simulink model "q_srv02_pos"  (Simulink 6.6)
settings: Solver=ode1  StartTime=0.0  StopTime=inf  FixedStep=0.002  RelTol=1e-3  AbsTol=1e-6
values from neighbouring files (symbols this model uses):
  K_AMP = 1    [setup_srv02_exp02_pos.m]    (also in setup_srv02_exp01_mdl.m; setup_srv02_exp03_spd.m)
  K_ENC = 0    [config_srv02.m]
  K_POT = -(352 * pi / 180 / 10)    (= -0.614355896702)    [config_srv02.m]
  K_TACH = -(1000 * 2 * pi / 60 / 1.5 / Kg)    [config_srv02.m]
  ki = -( -AmpMax + kp * e_ss ) / ti / e_ss    [d_i_design.m]    (also in setup_srv02_exp02_pos.m = 0; d_pi_design.m = wn^2*tau/K; setup_srv02_exp03_spd.m = 0)
  kp = wn^2/K*tau    [d_pv_design.m]    (also in setup_srv02_exp02_pos.m = 0; d_pi_design.m = (-1+2*zeta*wn*tau)/K; setup_srv02_exp03_spd.m = 0)
  kv = (-1+2*zeta*wn*tau)/K    [d_pv_design.m]    (also in setup_srv02_exp02_pos.m = 0)
  VMAX_AMP = 0    [config_srv02.m]
  VMAX_DAC = 10    [setup_srv02_exp02_pos.m]    (also in setup_srv02_exp01_mdl.m; setup_srv02_exp03_spd.m)
  wcf = 2 * pi * 50.0    (= 314.159265359)    [setup_srv02_exp02_pos.m]    (also in setup_srv02_exp03_spd.m)
  wcf_e = 2 * pi * 50.0    (= 314.159265359)    [setup_srv02_exp02_pos.m]    (also in setup_srv02_exp01_mdl.m = 157.079632679; setup_srv02_exp03_spd.m = 395.840674352)
  zetaf = 0.9    [setup_srv02_exp02_pos.m]    (also in setup_srv02_exp03_spd.m)
  zetaf_e = 0.9    [setup_srv02_exp02_pos.m]    (also in setup_srv02_exp01_mdl.m; setup_srv02_exp03_spd.m)
undefined symbols (not defined in the file or in its folder): HIL, qc_get_step_size, square
libraries: quarc_library x5

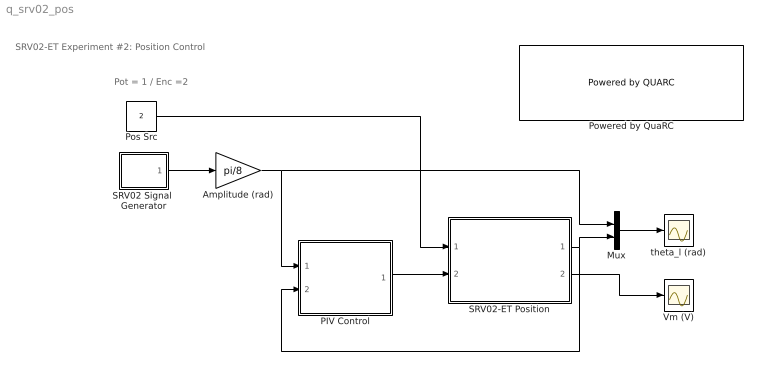
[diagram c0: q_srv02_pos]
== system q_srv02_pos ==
  note: SRV02-ET Experiment #2: Position Control
  note: Pot = 1 / Enc =2
  Amplitude (rad) : Gain  Gain=pi/8
  Mux : Mux  Inputs=2
  PIV Control : Subsystem
  Pos Src : Constant  Value=2
  Powered by QuaRC : quarc_library/Logos/Powered by QUARC  SystemSampleTime=-1
  SRV02 Signal  Generator : Subsystem  mask(QET Signal Generator){sig_type=square, a=1, f=0.4}
      mask prompts: sig_type "Signal Type"; a "Amplitude"; f "Frequency (Hz)"
      mask help: Generates a square, triangular, or sinusoidal waveform of a specified amplitude and frequency.
  SRV02-ET Position : Subsystem
  Vm (V) : Scope
  theta_l (rad) : Scope
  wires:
  Amplitude (rad)/1 -> Mux/1, PIV Control/1(theta_d (rad))
  SRV02-ET Position/1(theta_l (rad)) -> Mux/2, PIV Control/2(theta_l (rad))
  SRV02-ET Position/2(Vm (V)) -> Vm (V)/1
  Mux/1 -> theta_l (rad)/1
  PIV Control/1(u (V)) -> SRV02-ET Position/2(Vi (V))
  SRV02 Signal  Generator/1(out) -> Amplitude (rad)/1
  Pos Src/1 -> SRV02-ET Position/1(pos src)

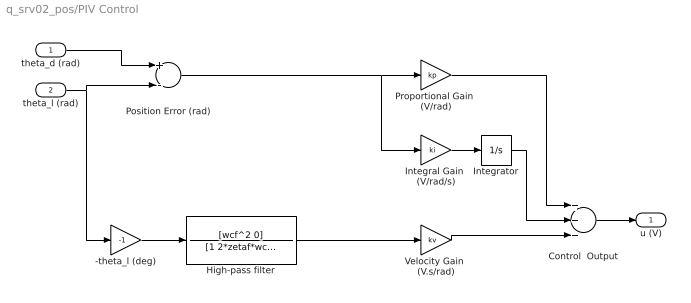
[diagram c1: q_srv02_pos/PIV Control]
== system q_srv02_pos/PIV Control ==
  theta_d (rad) : Inport
  theta_l (rad) : Inport  Port=2
  -theta_l (deg) : Gain  Gain=-1
  Control  Output : Sum  Inputs=+++  OutScaling=2^-10
  High-pass filter : TransferFcn  Numerator=[wcf^2 0]  Denominator=[1 2*zetaf*wcf wcf^2]
  Integral Gain  (V/rad/s) : Gain  Gain=ki
  Integrator : Integrator  LimitOutput=on  UpperSaturationLimit=VMAX_DAC  LowerSaturationLimit=-VMAX_DAC
  Position Error (rad) : Sum  Inputs=+-  OutScaling=2^-10
  Proportional Gain  (V/rad) : Gain  Gain=kp
  Velocity Gain  (V.s/rad) : Gain  Gain=kv
  u (V) : Outport
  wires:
  Integrator/1 -> Control  Output/2
  Velocity Gain  (V.s/rad)/1 -> Control  Output/3
  Integral Gain  (V/rad/s)/1 -> Integrator/1
  -theta_l (deg)/1 -> High-pass filter/1
  Position Error (rad)/1 -> Proportional Gain  (V/rad)/1, Integral Gain  (V/rad/s)/1
  theta_l (rad)/1 -> -theta_l (deg)/1, Position Error (rad)/2
  Control  Output/1 -> u (V)/1
  theta_d (rad)/1 -> Position Error (rad)/1
  Proportional Gain  (V/rad)/1 -> Control  Output/1
  High-pass filter/1 -> Velocity Gain  (V.s/rad)/1

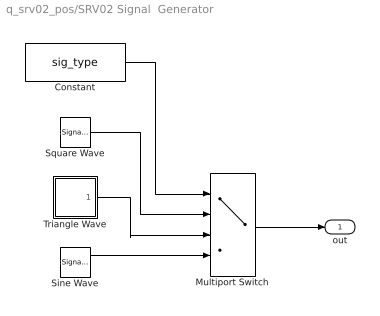
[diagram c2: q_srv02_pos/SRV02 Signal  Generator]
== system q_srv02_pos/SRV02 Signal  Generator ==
  Constant : Constant  Value=sig_type
  Multiport Switch : MultiPortSwitch  Inputs=3
  Sine Wave : SignalGenerator  Amplitude=a  Frequency=f
  Square Wave : SignalGenerator  WaveForm=square  Amplitude=a  Frequency=f
  Triangle Wave : Subsystem
  out : Outport
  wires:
  Constant/1 -> Multiport Switch/1
  Multiport Switch/1 -> out/1
  Sine Wave/1 -> Multiport Switch/4
  Triangle Wave/1(out) -> Multiport Switch/3
  Square Wave/1 -> Multiport Switch/2

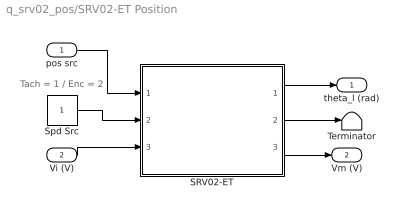
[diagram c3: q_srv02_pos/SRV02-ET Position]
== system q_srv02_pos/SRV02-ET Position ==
  note: Tach = 1 / Enc = 2
  pos src : Inport
  Vi (V) : Inport  Port=2
  SRV02-ET : Subsystem
  Spd Src : Constant
  Terminator : Terminator
  theta_l (rad) : Outport
  Vm (V) : Outport  Port=2
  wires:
  SRV02-ET/2(omega_l (rad/s)) -> Terminator/1
  Spd Src/1 -> SRV02-ET/2(spd src)
  pos src/1 -> SRV02-ET/1(pos src)
  SRV02-ET/1(theta_l (rad)) -> theta_l (rad)/1
  Vi (V)/1 -> SRV02-ET/3(Vi (V))
  SRV02-ET/3(Vm (V)) -> Vm (V)/1

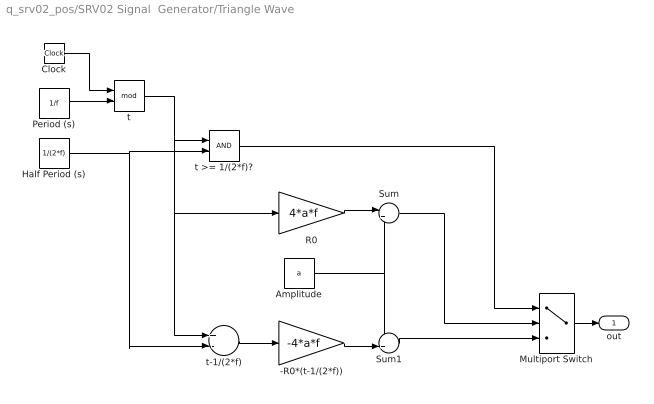
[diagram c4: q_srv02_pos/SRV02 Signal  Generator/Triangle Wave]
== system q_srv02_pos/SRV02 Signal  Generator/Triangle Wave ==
  -R0*(t-1/(2*f)) : Gain  Gain=-4*a*f
  Amplitude : Constant  Value=a
  Clock : Clock
  Half Period (s) : Constant  Value=1/(2*f)
  Multiport Switch : MultiPortSwitch  Inputs=2  zeroidx=on
  Period (s) : Constant  Value=1/f
  R0 : Gain  Gain=4*a*f
  Sum : Sum  Inputs=|+-
  Sum1 : Sum  Inputs=++|
  t : Math  Operator=mod
  t >= 1/(2*f)? : RelationalOperator  LogicOutDataTypeMode=Boolean
  t-1/(2*f) : Sum  Inputs=+-  OutScaling=2^-10
  out : Outport
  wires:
  Multiport Switch/1 -> out/1
  Clock/1 -> t/1
  Period (s)/1 -> t/2
  t/1 -> t >= 1/(2*f)?/1, R0/1, t-1/(2*f)/1
  Half Period (s)/1 -> t >= 1/(2*f)?/2, t-1/(2*f)/2
  t-1/(2*f)/1 -> -R0*(t-1/(2*f))/1
  R0/1 -> Sum/1
  Amplitude/1 -> Sum/2, Sum1/1
  -R0*(t-1/(2*f))/1 -> Sum1/2
  t >= 1/(2*f)?/1 -> Multiport Switch/1
  Sum/1 -> Multiport Switch/2
  Sum1/1 -> Multiport Switch/3

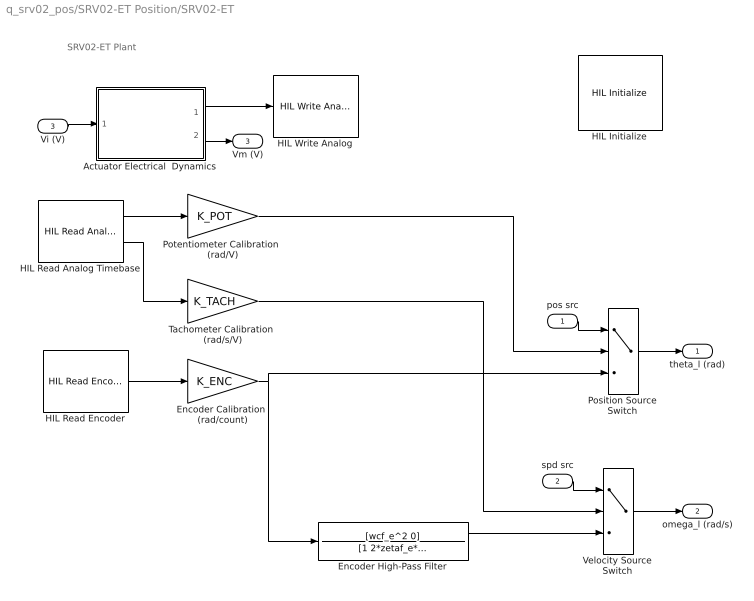
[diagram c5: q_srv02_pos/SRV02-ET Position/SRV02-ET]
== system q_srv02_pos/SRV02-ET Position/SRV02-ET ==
  note: SRV02-ET Plant
  pos src : Inport
  spd src : Inport  Port=2
  Vi (V) : Inport  Port=3
  Actuator Electrical  Dynamics : Subsystem
  Encoder Calibration  (rad/count) : Gain  Gain=K_ENC
  Encoder High-Pass Filter : TransferFcn  Numerator=[wcf_e^2 0]  Denominator=[1 2*zetaf_e*wcf_e wcf_e^2]
  HIL Initialize : quarc_library/Data Acquisition/Generic/Configuration/HIL Initialize  object_name=HIL-1  board_type=q8  board_number=0  exclusive=off  active=off  hardware_clocks=[0:1]  clock_modes=[0 0]  set_clock_params_at_start=on  set_clock_params_at_switch_in=off  analog_input_channels=[0:7]  analog_input_maximums=10  analog_input_minimums=-10  set_analog_input_params_at_start=off  set_analog_input_params_at_switch_in=off  analog_output_channels=[0:7]  analog_output_maximums=[10]  analog_output_minimums=[-10]  initial_analog_outputs=[0]  final_analog_outputs=[0]  watchdog_analog_outputs=0  set_analog_output_params_at_start=on  set_analog_output_params_at_switch_in=off  set_analog_outputs_at_start=on  set_analog_outputs_at_switch_in=off  set_analog_outputs_at_terminate=on  set_analog_outputs_at_switch_out=off  set_analog_outputs_on_watchdog=off  digital_input_channels=[]  digital_output_channels=[]  digital_output_configuration=[]  initial_digital_outputs=[1]  final_digital_outputs=[1]  watchdog_digital_outputs=[2]  set_digital_output_params_at_start=off  set_digital_output_params_at_switch_in=off  set_digital_outputs_at_start=on  set_digital_outputs_at_switch_in=off  set_digital_outputs_at_terminate=on  set_digital_outputs_at_switch_out=off  set_digital_outputs_on_watchdog=off  encoder_channels=[0:7]  quadrature=[4]  encoder_filter_frequency=(1/120e-9)/1  initial_encoder_counts=[0]  set_encoder_params_at_start=on  set_encoder_params_at_switch_in=off  set_encoder_counts_at_start=on  set_encoder_counts_at_switch_in=off  pwm_channels=[]  pwm_modes=[0]  pwm_frequency=(1/60e-9)/1024  pwm_configuration=[]  pwm_alignment=[]  pwm_polarity=[]  pwm_leading_deadband=[]  pwm_trailing_deadband=[]  initial_pwm_outputs=[0]  final_pwm_outputs=[0]  watchdog_pwm_outputs=[]  set_pwm_params_at_start=on  set_pwm_params_at_switch_in=off  set_pwm_outputs_at_start=on  set_pwm_outputs_at_switch_in=off  set_pwm_outputs_at_terminate=on  set_pwm_outputs_at_switch_out=off  set_pwm_outputs_on_watchdog=off  other_output_channels=[]  initial_other_outputs=[]  final_other_outputs=[]  watchdog_other_outputs=[]  set_other_outputs_at_start=off  set_other_outputs_at_switch_in=off  set_other_outputs_at_terminate=off  set_other_outputs_at_switch_out=off  set_other_outputs_on_watchdog=off
  HIL Read Analog Timebase : quarc_library/Data Acquisition/Generic/Timebases/HIL Read Analog Timebase  Tag=unassigned  object_name=HIL-1  clock=0  channels=[0,1]  samples_in_buffer=max(ceil(1/qc_get_step_size), 1)  active=on  vector_output=off
  HIL Read Encoder : quarc_library/Data Acquisition/Generic/Immediate I//O/HIL Read Encoder  Tag=unassigned  object_name=HIL-1  channels=0  sample_time=qc_get_step_size  active=on  vector_output=off  data_type_mode=Inherit via back propagation  data_type=double
  HIL Write Analog : quarc_library/Data Acquisition/Generic/Immediate I//O/HIL Write Analog  Tag=unassigned  object_name=HIL-1  channels=0  sample_time=-1  active=off  vector_input=off
  Position Source Switch : MultiPortSwitch  Inputs=2
  Potentiometer Calibration  (rad/V) : Gain  Gain=K_POT
  Tachometer Calibration  (rad/s/V) : Gain  Gain=K_TACH
  Velocity Source Switch : MultiPortSwitch  Inputs=2
  theta_l (rad) : Outport  InitialOutput=0
  omega_l (rad/s) : Outport  Port=2  InitialOutput=0
  Vm (V) : Outport  Port=3  InitialOutput=0
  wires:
  HIL Read Analog Timebase/2 -> Tachometer Calibration  (rad/s/V)/1
  HIL Read Encoder/1 -> Encoder Calibration  (rad/count)/1
  Encoder High-Pass Filter/1 -> Velocity Source Switch/3
  Potentiometer Calibration  (rad/V)/1 -> Position Source Switch/2
  spd src/1 -> Velocity Source Switch/1
  pos src/1 -> Position Source Switch/1
  Position Source Switch/1 -> theta_l (rad)/1
  Velocity Source Switch/1 -> omega_l (rad/s)/1
  HIL Read Analog Timebase/1 -> Potentiometer Calibration  (rad/V)/1
  Vi (V)/1 -> Actuator Electrical  Dynamics/1(Vi (V))
  Encoder Calibration  (rad/count)/1 -> Encoder High-Pass Filter/1, Position Source Switch/3
  Tachometer Calibration  (rad/s/V)/1 -> Velocity Source Switch/2
  Actuator Electrical  Dynamics/1(Vdaq (V)) -> HIL Write Analog/1
  Actuator Electrical  Dynamics/2(Vm (V)) -> Vm (V)/1

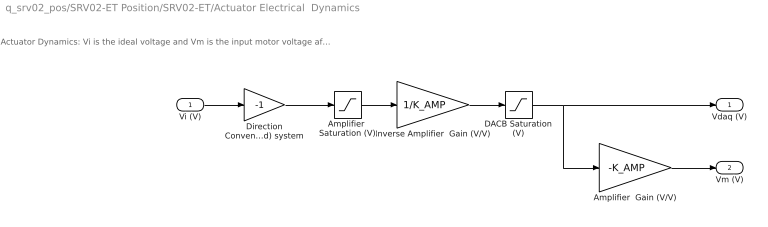
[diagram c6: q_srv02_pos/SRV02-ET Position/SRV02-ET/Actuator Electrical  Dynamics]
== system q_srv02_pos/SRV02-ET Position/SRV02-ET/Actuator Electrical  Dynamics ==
  note: Actuator Dynamics: Vi is the ideal voltage and Vm is the input motor voltage after going through the DAC and amplifier limitiations.
  Vi (V) : Inport
  Amplifier  Gain (V/V) : Gain  Gain=-K_AMP
  Amplifier  Saturation (V) : Saturate  UpperLimit=VMAX_AMP  LowerLimit=-VMAX_AMP
  DACB Saturation (V) : Saturate  UpperLimit=VMAX_DAC  LowerLimit=-VMAX_DAC
  Direction Convention: (Right-Hand) system : Gain  Gain=-1
  Inverse Amplifier  Gain (V/V) : Gain  Gain=1/K_AMP
  Vdaq (V) : Outport
  Vm (V) : Outport  Port=2
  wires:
  Vi (V)/1 -> Direction Convention: (Right-Hand) system/1
  Amplifier  Saturation (V)/1 -> Inverse Amplifier  Gain (V/V)/1
  Inverse Amplifier  Gain (V/V)/1 -> DACB Saturation (V)/1
  DACB Saturation (V)/1 -> Amplifier  Gain (V/V)/1, Vdaq (V)/1
  Amplifier  Gain (V/V)/1 -> Vm (V)/1
  Direction Convention: (Right-Hand) system/1 -> Amplifier  Saturation (V)/1
